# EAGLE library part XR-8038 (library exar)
Precision WAVEFORM GENERATOR
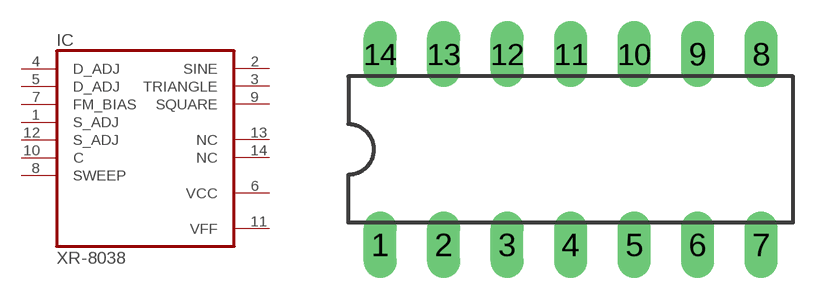
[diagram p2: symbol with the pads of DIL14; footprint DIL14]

Designator prefix IC

## XR-8038 (OC_FARNELL: unknown; OC_NEWARK: unknown)  [DIL14]
1  S_ADJ  in
2  SINE  out
3  TRIANGLE  out
4  D_ADJ  in
5  D_ADJ  in
6  VCC  pwr
7  FM_BIAS  in
8  SWEEP  in
9  SQUARE  out
10  C  in
11  VFF  pwr
12  S_ADJ  in
13  NC  nc
14  NC  nc

## Footprint DIL14 (pad centres in mm)
Dual In Line Package
drill 0.813 long: 1 -7.62,-3.81; 2 -5.08,-3.81; 3 -2.54,-3.81; 4 0,-3.81; 5 2.54,-3.81; 6 5.08,-3.81; 7 7.62,-3.81; 8 7.62,3.81; 9 5.08,3.81; 10 2.54,3.81; 11 0,3.81; 12 -2.54,3.81; 13 -5.08,3.81; 14 -7.62,3.81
